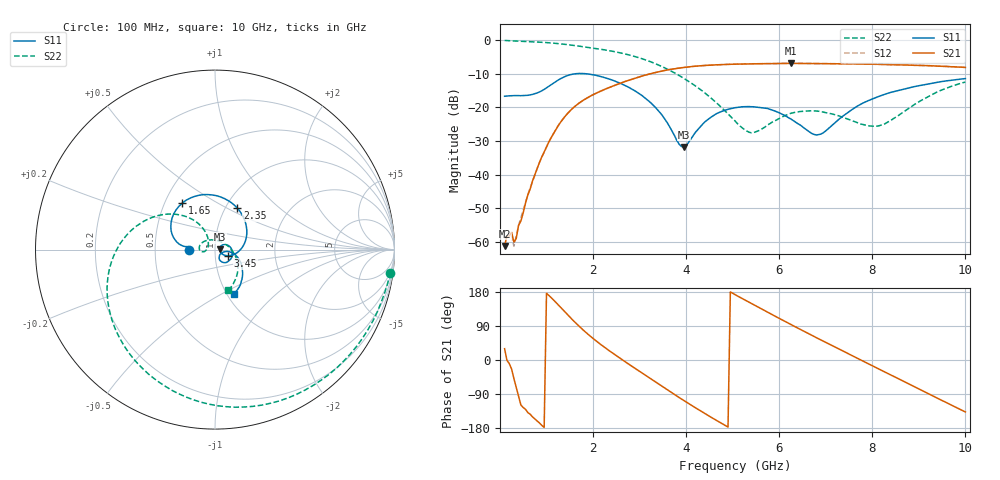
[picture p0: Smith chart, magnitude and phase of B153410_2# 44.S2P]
!  2-Port S-parameters saved by WinCal
! VAR MeasName=S-Parameters (CALIBRATED_DATA) read from VNA (N5245A)
! VAR MeasDate=2016-12-23 10:01:37
! VAR NAME=B153410_2# 44
! VAR FILENAME=B153410_2# 44.S2P
! VAR DATE=2016-12-23 10:01:37
! VAR PHYS_PORTS=1,2
# Hz S DB R 50
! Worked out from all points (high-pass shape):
!   199 points, 100 MHz to 10 GHz, reference 50 ohm
!   highest |S21| = -6.94 dB at 6.25 GHz (marker M1); lowest = -61.2 dB at 100 MHz (marker M2)
!   |S21| within 3 dB of the highest: 3.255 GHz to end of sweep
!   lowest |S11| = -31.8 dB at 3.95 GHz (marker M3), VSWR 1.05, Z = 52.6 + j0.257 ohm
!   |S11| at or under -10 dB: start of sweep to 1.64 GHz; 1.831 GHz to end of sweep
!   |S22| runs from -27.6 to -0.1 dB; largest |S21 - S12| = 0.0031
!   S11 on the Smith chart (normalised r, x): 100 MHz: 0.75, -0.00; 1.65 GHz: 0.61, +0.35; 2.35 GHz: 1.13, +0.56; 3.45 GHz: 1.16, -0.08; 10 GHz: 1.08, -0.57
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1e8  -16.71 -179.7  -61.24 29.8  -58.91 31.7  -0.13 -7.5
2.5e8  -16.54 177.3  -57.14 -23.7  -58.24 -42.2  -0.25 -17.6
3e8  -16.49 176.3  -60.04 -49.0  -61.26 -36.5  -0.28 -21.0
6e8  -16.42 173.6  -46.00 -138.9  -45.90 -140.3  -0.46 -40.8
8.5e8  -15.43 174.1  -36.35 -166.4  -36.37 -166.9  -0.63 -57.1
1.25e9  -11.91 160.4  -25.48 146.0  -25.49 146.2  -1.06 -82.7
1.65e9  -9.98 125.1  -19.28 95.1  -19.28 95.1  -1.72 -106.9
1.75e9  -9.94 115.6  -18.26 83.5  -18.30 83.4  -1.91 -112.6
2.35e9  -11.60 61.9  -14.09 24.3  -14.10 24.5  -3.17 -145.9
3.4e9  -20.94 -21.9  -9.47 -62.8  -9.45 -62.8  -7.39 158.3
3.45e9  -21.75 -25.0  -9.30 -67.0  -9.30 -66.8  -7.69 156.0
3.95e9  -31.79 5.4  -8.16 -106.8  -8.14 -106.7  -11.38 134.7
4.45e9  -23.81 26.5  -7.51 -144.8  -7.52 -144.8  -16.25 120.8
5.05e9  -20.12 -9.2  -7.17 172.5  -7.19 172.7  -24.04 126.8
5.45e9  -19.84 -32.5  -7.05 145.7  -7.06 145.7  -27.51 164.0
6.25e9  -23.46 -65.1  -6.94 93.8  -6.95 93.8  -21.77 -174.0
6.7e9  -27.77 -51.3  -6.95 65.2  -6.96 65.3  -21.06 169.8
6.95e9  -27.54 -25.7  -7.00 49.6  -7.01 49.7  -21.41 158.7
7.55e9  -20.81 -9.8  -7.09 12.5  -7.10 12.6  -23.88 123.7
8.35e9  -15.77 -27.5  -7.32 -36.6  -7.29 -36.3  -24.26 35.4
9.15e9  -13.20 -46.2  -7.59 -85.4  -7.59 -85.3  -17.19 -27.8
1e10  -11.45 -66.7  -8.15 -137.2  -8.12 -136.8  -12.48 -71.6
